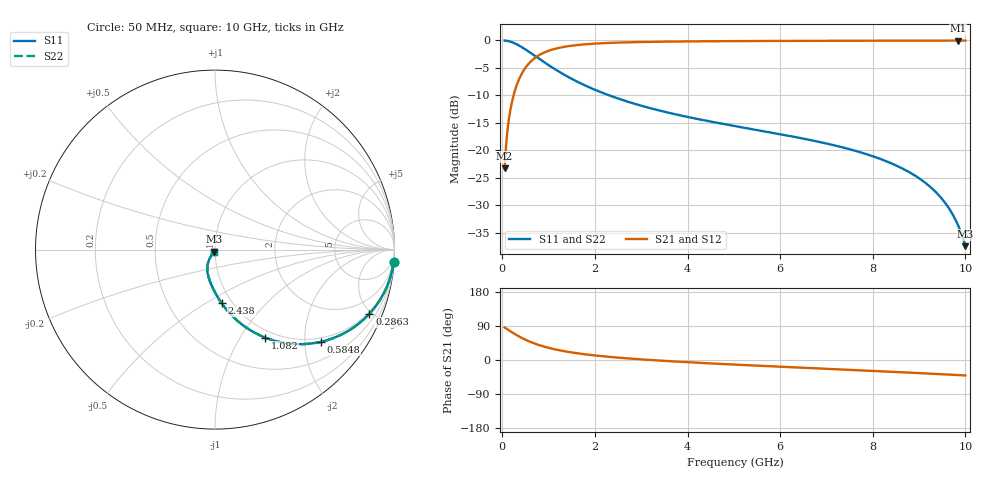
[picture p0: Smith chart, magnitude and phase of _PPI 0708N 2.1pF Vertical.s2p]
! S-Parameter data specifications (vertical orientation):
! Substrate: 40-mil Rogers 3003C, Substrate thickness, H=1.016mm, Dielectric constant, Er=3, Conductor thickness, T_mtl=0.043mm, Loss Tangent, Tand=0.003
! PCB Mounting Pad Footprint: Pad width, PadW=2.54mm , Pad length, PadL=0.51mm , Pad gap, PadG (edge-to-edge)=0.71mm , Reference planes=1.73mm apart
! Created Tue Jan 16 08:44:20 2018
# GHz S MA R 50
! 2 Port Network Data from SP1.SP block
! freq  magS11  angS11  magS21  angS21  magS12  angS12  magS22  angS22
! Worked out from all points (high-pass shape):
!   801 points, 50 MHz to 10 GHz, reference 50 ohm
!   highest |S21| = -0.04 dB at 9.838 GHz (marker M1); lowest = -23.3 dB at 50 MHz (marker M2)
!   |S21| within 3 dB of the highest: 731.8 MHz to end of sweep
!   lowest |S11| = -37.5 dB at 10 GHz (marker M3), VSWR 1.03, Z = 49.5 - j1.22 ohm
!   |S11| at or under -10 dB: 2.301 GHz to end of sweep
!   |S22| runs from -37.5 to 0.0 dB; largest |S21 - S12| = 0
!   S11 on the Smith chart (normalised r, x): 50 MHz: 1, -28; 286.3 MHz: 0.90, -4.85; 584.8 MHz: 0.90, -2.38; 1.082 GHz: 0.90, -1.29; 2.438 GHz: 0.89, -0.59; 10 GHz: 0.99, -0.02
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0.05  0.9977 -4.1  0.0681 85.9  0.0681 85.9  0.9977 -4.1
0.124625  0.9858 -10.2  0.1677 79.8  0.1677 79.8  0.9858 -10.2
0.1619375  0.9764 -13.2  0.2158 76.8  0.2158 76.8  0.9764 -13.2
0.224125  0.9562 -18.0  0.2925 72.0  0.2925 72.0  0.9562 -18.0
0.2863125  0.9314 -22.6  0.3638 67.4  0.3638 67.4  0.9314 -22.6
0.423125  0.8661 -31.8  0.4995 58.2  0.4995 58.2  0.8661 -31.8
0.5848125  0.7823 -41.1  0.6225 48.9  0.6225 48.9  0.7823 -41.1
0.821125  0.6678 -51.7  0.7437 38.3  0.7437 38.3  0.6678 -51.7
1.082313  0.5645 -60.3  0.8247 29.6  0.8247 29.6  0.5645 -60.3
1.368375  0.4781 -67.3  0.8774 22.6  0.8774 22.6  0.4781 -67.3
1.716625  0.4013 -73.7  0.9149 16.1  0.9149 16.1  0.4013 -73.7
2.438  0.3014 -82.9  0.9522 6.9  0.9522 6.9  0.3014 -82.9
3.370812  0.2308 -91.0  0.9715 -1.3  0.9715 -1.3  0.2308 -91.0
5.025  0.1656 -101.5  0.9842 -12.2  0.9842 -12.2  0.1656 -101.5
6.691625  0.1227 -110.5  0.9899 -21.5  0.9899 -21.5  0.1227 -110.5
7.624437  0.09862 -115.1  0.9922 -26.7  0.9922 -26.7  0.09862 -115.1
8.345812  0.07759 -118.5  0.9937 -30.7  0.9937 -30.7  0.07759 -118.5
8.868187  0.06019 -120.6  0.9945 -33.7  0.9945 -33.7  0.06019 -120.6
9.278625  0.04481 -121.6  0.9951 -36.2  0.9951 -36.2  0.04481 -121.6
9.602  0.03142 -121.2  0.9953 -38.2  0.9953 -38.2  0.03142 -121.2
9.838313  0.02087 -118.6  0.9954 -39.7  0.9954 -39.7  0.02087 -118.6
10  0.01335 -112.5  0.9953 -40.8  0.9953 -40.8  0.01335 -112.5
